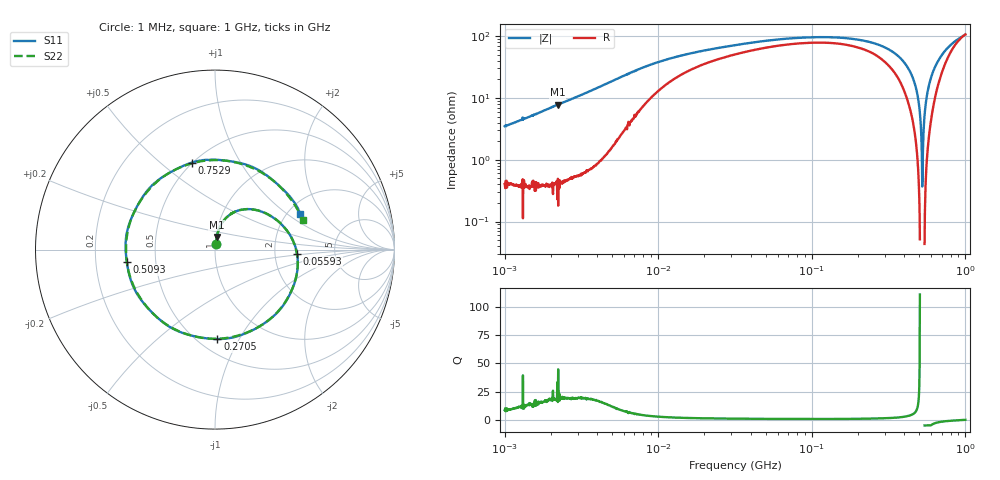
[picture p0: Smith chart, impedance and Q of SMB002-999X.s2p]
!s-Parameter Generated by FASTRON Sdn. Bhd.
!FASTRON P/N : SMB/002-999X
!Vector Network Analyser E5071C,MY46733604,B.14.02
!Date: Mon Jul 31 13:21:32 2023
!Data & Calibration Information:
!Freq	S11:SOLT2(ON)	S21:SOLT2(ON)	S12:SOLT2(ON)	S22:SOLT2(ON)
!PortZ  Port1:50+j0  Port2:50+j0
!When reading, reference impedance value at option line is always used.
! Remarks : This data is being provided solely for informational purposes.
# Hz S dB R 50
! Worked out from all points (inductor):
!   1601 points, 1 MHz to 1 GHz, reference 50 ohm
!   read as one part in series: L = 546 nH near 1.041 MHz
!   highest Q = 19.7 at 2.213 MHz (marker M1), where L = 559 nH
!   self-resonance near 524.5 MHz
!   S11 on the Smith chart (normalised r, x): 1 MHz: 1.01, +0.07; 55.93 MHz: 2.68, -0.16; 270.5 MHz: 0.62, -0.82; 509.3 MHz: 0.34, -0.06; 752.9 MHz: 0.50, +0.64; 1 GHz: 2.33, +1.26
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1000000  -29.68 79.0  -0.03 -2.1  -0.04 -2.1  -29.84 79.2
1459136  -26.76 82.9  -0.04 -3.2  -0.04 -3.1  -27.13 81.3
2213160  -22.98 82.0  -0.04 -4.8  -0.04 -4.8  -22.91 82.8
3167252  -19.85 80.2  -0.10 -6.9  -0.10 -6.9  -19.87 80.1
5629542  -14.46 70.4  -0.37 -12.8  -0.36 -12.8  -14.46 70.4
1.002882e7  -10.48 48.7  -1.42 -19.7  -1.42 -19.7  -10.46 48.5
3.163788e7  -7.53 12.9  -3.90 -26.2  -3.90 -26.2  -7.53 12.8
5.592793e7  -6.78 -3.0  -4.82 -31.9  -4.81 -31.9  -6.78 -3.4
1.00144e8  -6.35 -24.4  -5.50 -43.5  -5.50 -43.5  -6.34 -24.7
1.70249e8  -6.12 -52.0  -5.83 -64.4  -5.82 -64.3  -6.13 -52.8
2.705257e8  -6.05 -88.4  -5.96 -96.5  -5.95 -96.5  -6.07 -89.7
3.171813e8  -6.08 -105.3  -5.99 -111.9  -5.99 -111.9  -6.08 -106.3
4.023222e8  -6.09 -135.1  -6.01 -140.5  -6.00 -140.5  -6.09 -136.4
5.092527e8  -6.09 -172.0  -6.04 -176.8  -6.03 -176.8  -6.10 -173.6
5.662042e8  -6.02 168.8  -6.05 163.9  -6.04 163.9  -6.08 166.8
6.219895e8  -6.08 149.5  -6.07 144.7  -6.08 144.8  -6.09 147.5
6.804311e8  -6.02 129.9  -6.09 124.7  -6.09 124.8  -6.06 127.4
7.528988e8  -5.99 104.9  -6.14 99.9  -6.14 99.9  -6.06 102.6
8.0822e8  -6.03 86.3  -6.17 80.6  -6.17 80.7  -6.04 83.4
8.635411e8  -5.94 67.7  -6.22 61.6  -6.22 61.6  -6.01 64.7
9.373027e8  -5.92 42.8  -6.33 35.6  -6.33 35.7  -5.94 39.7
1e9  -5.78 22.7  -6.52 13.3  -6.51 13.5  -5.76 18.4
